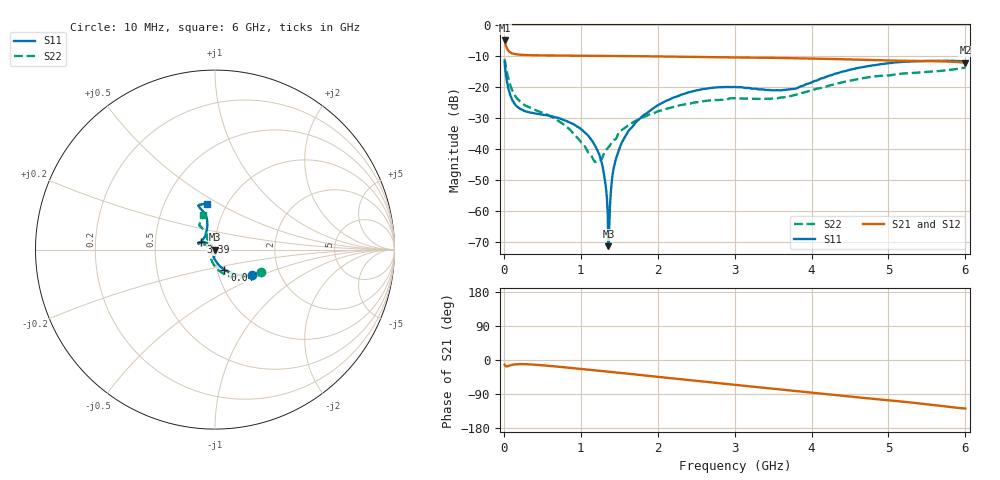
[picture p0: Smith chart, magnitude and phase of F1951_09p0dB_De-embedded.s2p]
! Integrated Device Technology
! Corporate Headquarters
! 6024 Silver Creek Valley Road
! San Jose, CA 95138  USA
! Phone:  1-408-284-8200
! Toll Free:  1-800-223-1366
! Webpage:  http://www.idt.com/
! Timing and RF Division
! 515 Groton Road, Suite 102
! Westford, MA 01886-6024
! Device:  F1951
! Description: 6-bit 0.5 dB Digital Step Attenuator
! Frequency:  100.0 -  4000.00 MHz
! Package:  4x4 mm Thin QFN Plastic Package: 24 pin
! Ports:  2 RF, 6 DC
!  Pin  1  = NC
!  Pin  2  = RF1  =  Port 1
!  Pin  3  = GND
!  Pin  4  = NC
!  Pin  5  = Serial Data Out (SDO)
!  Pin  6  = NC
!  Pin  7  = Reset Bar ( RSTb)
!  Pin  8  = Clock (CLK)
!  Pin  9  = Chip Select Bar (CSb)
!  Pin 10  = NC
!  Pin 11  = Serial Data In (SDI)
!  Pin 12  = NC
!  Pin 13  = NC
!  Pin 14  = VDD
!  Pin 15  = NC
!  Pin 16  = GND
!  Pin 17  = RF2  =  Port 2
!  Pin 18  = NC
!  Pin 19  = GND
!  Pin 20  = GND
!  Pin 21  = GND
!  Pin 22  = GND
!  Pin 23  = GND
!  Pin 24  = GND
! State:  18
! Atten State:  9.0 dB
! Voltage:  +3.30 Volts
! Current:  0.474 mA
! Data:  The device was measured on a F195X evaluation board which has
!  individual transmission lines to the RF pins.  Data was collected
!  de-embedded using a Automatic Fixture Removal [AFR] (Keysight Technologies).
!  The reference plane is the edge of the package pin.
! Misc:  Lot Code  1225BCA
!  Action Tracker AT0399
! Date Measured:  2018-09-13
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# GHz S dB R 50
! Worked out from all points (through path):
!   600 points, 10 MHz to 6 GHz, reference 50 ohm
!   highest |S21| = -5.01 dB at 10 MHz (marker M1); lowest = -12.2 dB at 6 GHz (marker M2)
!   group delay of S21, straight-line fit = 56.8 ps
!   lowest |S11| = -71.5 dB at 1.36 GHz (marker M3), VSWR 1.00, Z = 50 - j0.021 ohm
!   |S11| at or under -10 dB: start of sweep to end of sweep
!   |S22| runs from -44.3 to -11.0 dB; largest |S21 - S12| = 0.00054
!   S11 on the Smith chart (normalised r, x): 10 MHz: 1.44, -0.44; 40 MHz: 1.08, -0.25; 3.39 GHz: 0.85, +0.07; 6 GHz: 0.81, +0.43
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0.01  -12.02 -34.7  -5.01 -12.5  -5.01 -12.5  -11.00 -25.7
0.04  -18.17 -64.9  -7.54 -16.8  -7.53 -16.8  -15.18 -60.2
0.1  -23.71 -85.5  -9.10 -13.1  -9.10 -13.1  -20.60 -90.1
0.2  -26.91 -98.7  -9.59 -10.9  -9.59 -10.9  -24.47 -110.2
0.76  -30.59 -91.9  -9.89 -18.7  -9.89 -18.8  -31.84 -124.4
1.01  -33.78 -80.9  -9.96 -23.7  -9.96 -23.7  -38.07 -128.0
1.17  -38.34 -76.2  -9.98 -26.8  -9.98 -26.8  -43.78 -161.7
1.25  -42.57 -74.0  -9.99 -28.5  -9.99 -28.5  -43.56 162.8
1.3  -48.02 -74.0  -9.99 -29.5  -10.00 -29.5  -41.62 140.4
1.34  -55.97 -81.1  -10.00 -30.4  -10.01 -30.4  -40.10 135.8
1.36  -71.46 -128.0  -10.01 -30.8  -10.01 -30.9  -39.57 132.0
1.38  -58.31 117.1  -10.01 -31.2  -10.01 -31.2  -38.91 127.7
1.44  -44.92 120.9  -10.04 -32.5  -10.04 -32.5  -37.05 123.7
1.54  -37.68 121.2  -10.05 -34.5  -10.05 -34.5  -33.84 120.0
1.72  -31.31 126.8  -10.08 -38.4  -10.09 -38.4  -30.89 121.1
2.01  -25.82 137.7  -10.17 -44.6  -10.17 -44.6  -27.83 129.6
2.49  -21.18 151.4  -10.32 -54.8  -10.32 -54.8  -25.02 145.7
3.01  -20.03 159.5  -10.50 -65.7  -10.50 -65.7  -23.65 152.7
3.39  -20.95 151.7  -10.59 -73.6  -10.60 -73.6  -23.88 142.4
4.01  -18.42 112.1  -10.84 -86.7  -10.84 -86.7  -21.11 119.9
5.01  -12.36 109.6  -11.51 -106.4  -11.51 -106.4  -16.30 122.7
6  -11.84 100.6  -12.18 -128.0  -12.18 -128.0  -13.80 108.5
